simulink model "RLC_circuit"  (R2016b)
settings: Solver=VariableStepAuto  StartTime=0.0  StopTime=10.0  MaxStep=0.001  RelTol=1e-3

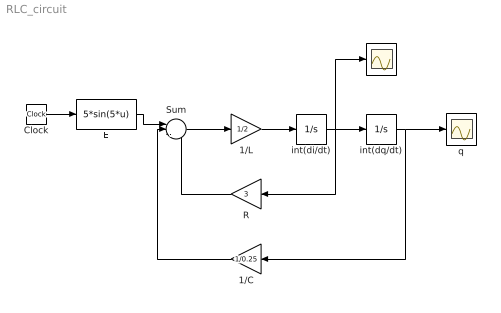
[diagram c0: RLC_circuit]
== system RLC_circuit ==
  1/C : Gain  Gain=1/0.25
  1/L : Gain  Gain=1/2
  Clock : Clock
  E : Fcn  Expr=5*sin(5*u)
  R : Gain  Gain=3
  Sum : Sum  Inputs=|+--
  i : Scope
  int(di/dt) : Integrator
  int(dq/dt) : Integrator
  q : Scope
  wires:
  Clock/1 -> E/1
  E/1 -> Sum/1
  Sum/1 -> 1/L/1
  1/L/1 -> int(di/dt)/1
  int(di/dt)/1 -> i/1, R/1, int(dq/dt)/1
  int(dq/dt)/1 -> q/1, 1/C/1
  R/1 -> Sum/3
  1/C/1 -> Sum/2
